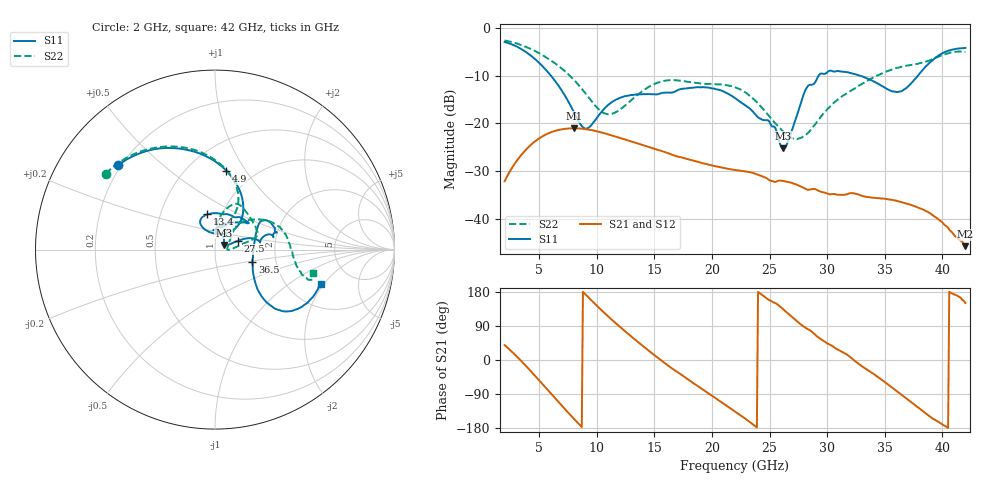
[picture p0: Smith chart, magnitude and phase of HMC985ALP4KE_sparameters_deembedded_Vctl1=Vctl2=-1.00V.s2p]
!s2p File: Measurements: S11, S21, S12, S22
# GHz S dB R 50.0
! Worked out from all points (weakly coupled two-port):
!   401 points, 2 GHz to 42 GHz, reference 50 ohm
!   highest |S21| = -21.02 dB at 8 GHz (marker M1); lowest = -45.8 dB at 42 GHz (marker M2)
!   lowest |S11| = -25.3 dB at 26.2 GHz (marker M3), VSWR 1.12, Z = 55 + j2.78 ohm
!   |S11| at or under -10 dB: 6.028 GHz to 29.25 GHz (23.23 GHz wide, 132 % of centre); 32.86 GHz to 37.86 GHz (4.999 GHz wide, 14.1 % of centre)
!   |S22| runs from -23.3 to -2.6 dB; largest |S21 - S12| = 0.0002
!   S11 on the Smith chart (normalised r, x): 2 GHz: 0.19, +0.36; 4.9 GHz: 0.75, +0.82; 13.4 GHz: 0.85, +0.35; 27.5 GHz: 1.28, +0.12; 36.5 GHz: 1.51, -0.21; 42 GHz: 3.01, -1.86
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2  -2.90 138.7  -32.12 39.3  -32.12 39.3  -2.59 145.2
3.4  -4.34 111.4  -26.76 -1.2  -26.76 -1.2  -3.52 122.5
4.9  -7.06 81.7  -23.30 -50.3  -23.30 -50.3  -5.14 99.2
6.3  -10.84 56.7  -21.63 -98.1  -21.64 -98.1  -7.25 79.7
8  -17.56 49.2  -21.02 -154.6  -21.03 -154.6  -10.81 63.4
8.7  -20.56 67.5  -21.10 -176.9  -21.11 -176.9  -12.74 61.0
9.3  -20.87 93.6  -21.30 164.5  -21.30 164.5  -14.57 61.9
10.9  -16.31 119.7  -22.23 117.5  -22.24 117.5  -18.05 77.9
13.4  -13.93 102.0  -24.09 51.8  -24.10 51.8  -14.27 80.4
15.4  -13.79 75.0  -25.62 3.8  -25.62 3.7  -11.35 68.4
18.9  -12.42 39.1  -28.15 -71.6  -28.16 -71.6  -11.57 41.3
22  -14.67 54.9  -29.75 -135.5  -29.76 -135.5  -12.42 17.2
24.9  -19.38 90.8  -31.75 159.3  -31.76 159.3  -18.27 7.7
26.2  -25.26 27.5  -32.09 133.0  -32.09 132.9  -21.78 -0.7
27.5  -17.39 20.7  -33.00 99.1  -33.01 99.2  -23.19 5.6
28.7  -11.87 9.4  -33.76 73.9  -33.75 74.0  -20.98 27.6
31  -9.02 20.3  -34.98 26.2  -35.01 26.3  -14.82 47.9
33.3  -10.38 31.6  -35.37 -21.8  -35.36 -22.0  -11.35 38.2
35.4  -13.00 10.6  -35.96 -67.2  -35.98 -67.3  -8.89 23.9
36.5  -13.20 -17.9  -36.55 -92.7  -36.58 -92.8  -8.08 15.4
39.6  -5.90 -42.5  -40.00 -162.2  -40.04 -163.1  -6.07 -15.3
42  -4.16 -17.9  -45.76 150.3  -45.82 150.0  -5.01 -13.5
